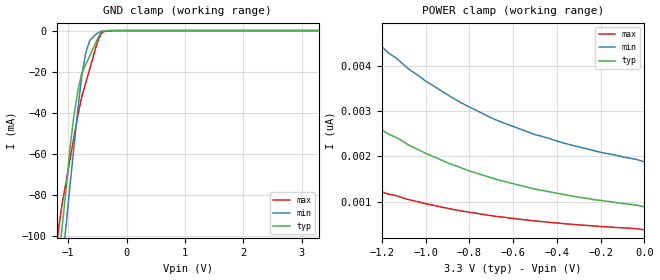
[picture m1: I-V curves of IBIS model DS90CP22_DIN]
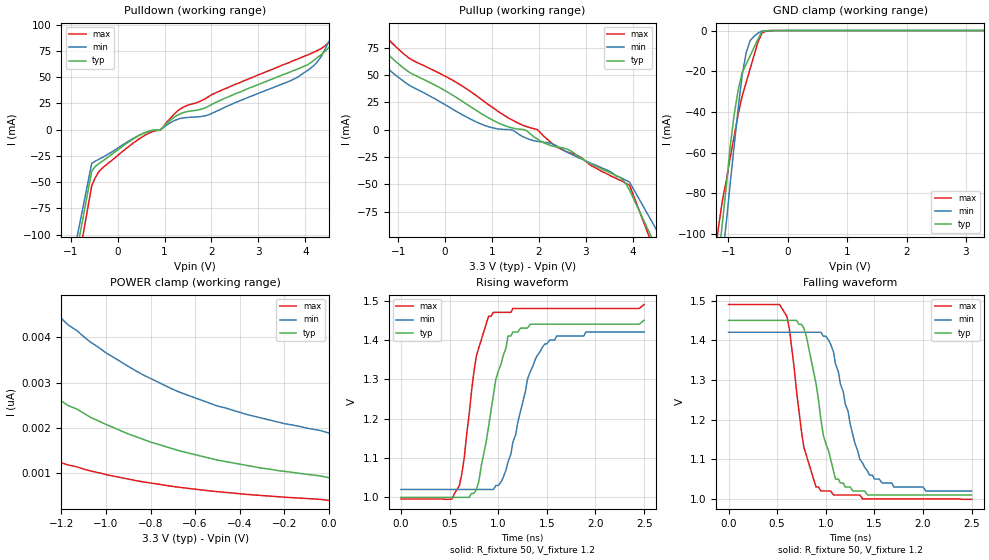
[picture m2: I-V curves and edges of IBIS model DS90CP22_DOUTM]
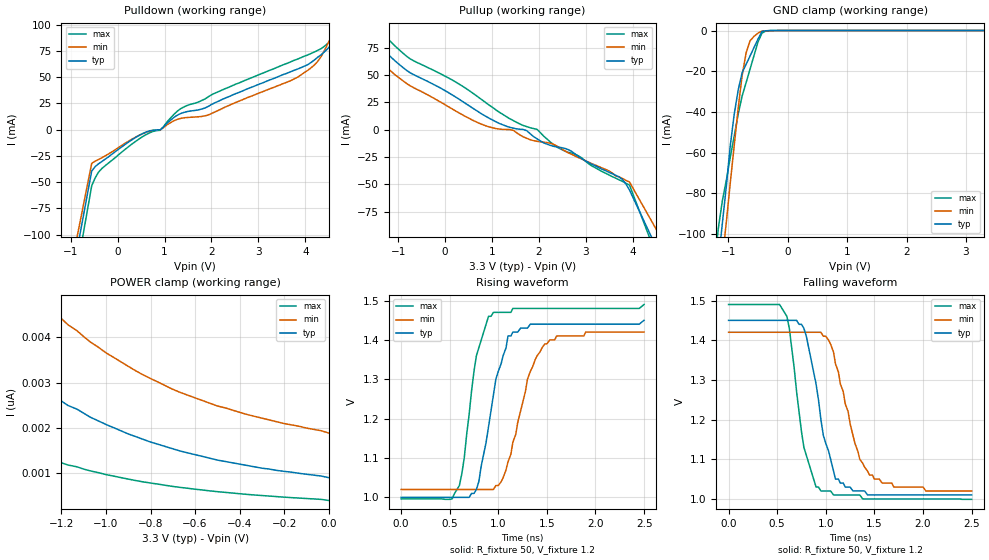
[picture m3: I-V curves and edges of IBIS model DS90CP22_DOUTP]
|   National Semiconductor Corporation
|   IBIS Model of DS90CP22MT
|   2 X 2 800 Mbps LVDS Crosspoint Switch
|   16 Lead TSSOP Package
[IBIS Ver]   3.2
[Comment Char]   |_char
[File name]   ds90cp22mt.ibs
[File Rev]   1.0
[Date]   12/19/03
[Source]
SPICE to IBIS Translation
[Notes]
Created by DG
Rev. 1.0:
- All data from ds90cp22m8 with updated package parasitics for TSSOP package
[Disclaimer]
(C) Copyright National Semiconductor Corporation 2002
   All rights reserved
   National Semiconductor Corporation hereby grants
the user of this IBIS model a non-exclusive, nontransferable
license to use this IBIS model under the following terms.
Before using this IBIS model, the user should read this
license.  If the user does not accept these terms,  the
IBIS model should be returned to National within 30 days.
   The user is granted this license only to use the
IBIS model and is not granted rights to sell, load, rent,
lease or license the IBIS model in whole or in part, or in
modified form to anyone other than user. User may modify
the IBIS model to suit its specific applications but rights
to derivative works and such modifications shall belong to
National.
   This IBIS model is provided on an "AS IS" basis and
National makes absolutely no warranty with respect to the
information contained herein.NATIONAL DISCLAIMS AND CUSTOMER
WAIVES ALL WARRANTIES, EXPRESS OR IMPLIED, INCLUDING
WARRANTIES OF MERCHANTABILITY OR FITNESS FOR A PARTICULAR
PURPOSE. The entire risk as to quality and performance is
with the Customer. ACCORDINGLY, IN NO EVENT SHALL THE
COMPANY BE LIABLE FOR ANY DAMAGES, WHETHER IN CONTRACT OR
TORT,INCLUDING ANY LOST PROFITS OR OTHER INCIDENTAL,
CONSEQUENTIAL, EXEMPLARY, OR PUNITIVE DAMAGES ARISING OUT
OF THE USE OR APPLICATION OF THE IBIS model provided in
this package.Further, National reserves the right to make
changes without notice to any product herein to improve
reliability, function, or design. National does not convey
any license under patent rights or any other intellectual
property rights, including those of third parties.
   National is not obligated to provide maintenance or support
for the licensed IBIS model.
Contact National at ATTN:INTERFACE APPLICATIONS/IBIS MODELS.
5 Foden Road, M/S 03-03, South Porltand, ME 04106
(207) 541-6031
[Copyright]
(c) Copyright 2002 National Semiconductor Corp.
[Component]   DS90CP22MT
Si_location Pin
Timing_location Pin
[Manufacturer]   National Semiconductor Corp.
[Package]
|   TYP   MIN   MAX
R_pkg   91m   78m   115m
L_pkg   2.49n   2.15n   3.12n
C_pkg   0.086p   0.076p   0.109p
[Pin]   signal_name   model_name   R_pin   L_pin   C_pin
1   SEL1   DS90CP22_CONTROL  113m   3.053n   .108p
2   SEL0   DS90CP22_CONTROL   91m   2.494n   .083p
3   IN0+   DS90CP22_DIN   80m   2.218n   .079p
4   IN0-   DS90CP22_DIN   78m   2.157n   .076p
5   VDD   POWER   79m   2.183n   .077p
6   IN1+   DS90CP22_DIN   84m   2.318n   .078p
7   IN1-   DS90CP22_DIN   93m   2.550n   .083p
8   NC   NC   108m   2.984n   .107p
9   NC   NC   115m   3.121n   .109p
10   OUT1-   DS90CP22_DOUTM   93m   2.551n   .083p
11   OUT1+   DS90CP22_DOUTP   81m   2.237n   .079p
12   GND   GND   78m   2.152n   .076p
13   OUT0-   DS90CP22_DOUTM   79m   2.173n   .076p
14   OUT0+   DS90CP22_DOUTP   83m   2.291n   .078p
15   EN1   DS90CP22_CONTROL   90m   2.480n   .083p
16   EN0   DS90CP22_CONTROL  106m   2.914n   .106p
[Diff Pin] inv_pin vdiff   tdelay_typ tdelay_min tdelay_max
| The '+' pin is Diff_pin and the '-' pin is the inv_pin
| Vth/Vtl of Reciever = 100mv
3   4   100mv   0   0   0
6   7   100mv   0   0   0
11   10   0   0   0   0
14   13   0   0   0   0
| Models and submodels in the file (4): DS90CP22_DIN (Input), DS90CP22_DOUTM (3-state), DS90CP22_DOUTP (3-state), DS90CP22_CONTROL (Input)
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[Model]   DS90CP22_DIN
Model_type Input
Vinh=.1
Vinl=-.1
C_comp   2.49pF   2.49pF   2.49pF
[Temperature Range] 25   85   -40
[Voltage Range]   3.3   3.0   3.6
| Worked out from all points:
|   GND clamp passes 1 mA (typ) near -0.44 V on its own axis
[GND Clamp]
|V(groundclamp)   I(typ)   I(min)   I(max)
-3.3V     -803mA     -823mA     -782mA
-1.17V    -114mA     -132mA     -97.7mA
-1.1V     -94.8mA    -112mA     -83.7mA
-1.03V    -75.7mA    -93.4mA    -73.1mA
-967mV    -56.7mA    -75mA      -62.4mA
-900mV    -41.1mA    -56.5mA    -51.8mA
-833mV    -29.2mA    -38.1mA    -41.1mA
-767mV    -20.7mA    -22.1mA    -32.2mA
-700mV    -16.6mA    -11mA      -25.6mA
-633mV    -12.5mA    -5.01mA    -18.9mA
-433mV    -470uA     -263uA     -1.31mA
3.3V      923pA      1.92nA     295pA
[POWER Clamp]
|Vtable   I(typ)   I(min)   I(max)
-3.3V     38.3nA     45.4nA     26.1nA
-2.17V    9.04nA     12.9nA     4.91nA
-2.13V    8.68nA     12.5nA     4.68nA
-2.07V    7.94nA     11.6nA     4.23nA
-1.87V    6.06nA     9.14nA     3.12nA
-1.7V     4.86nA     7.56nA     2.44nA
-1.47V    3.61nA     5.85nA     1.75nA
-1.27V    2.82nA     4.74nA     1.34nA
-1V       2.07nA     3.66nA     958pA
-700mV    1.53nA     2.85nA     695pA
-500mV    1.28nA     2.48nA     579pA
0V        889pA      1.88nA     383pA
[Model]   DS90CP22_DOUTM
Model_type 3-state
Enable Active-High
Polarity Inverting
Vref=1.2
Vmeas=1.2
Rref=50   | 100 Ohms Across Outputs OUTP and OUTM
Cref=5p
C_comp   3.493pF   3.493pF   3.493pF
[Temperature Range] 25   85   -40
[Voltage Range]   3.3   3.0   3.6
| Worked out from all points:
|   slope of the pulldown table from 0 to 0.495 V, typ, clamps not added: 33.8 ohm
|   slope of the pullup table from 0 to 0.495 V, typ, clamps not added: 37.2 ohm
|   GND clamp passes 1 mA (typ) near -0.44 V on its own axis
|   falling waveform, R_fixture 50, V_fixture 1.2: 20-80 % time 212ps typ, 250ps min, 172ps max; typ from 1.45 V to 1.01 V
|   rising waveform, R_fixture 50, V_fixture 1.2: 20-80 % time 217ps typ, 250ps min, 167ps max; typ from 1 V to 1.45 V
[Pullup]
|Vtable   I(typ)   I(min)   I(max)
-3.3V     282mA      249mA      331mA
-1.69V    113mA      101mA      125mA
-1.62V    104mA      93.1mA     115mA
-1.48V    87.5mA     77.5mA     98.1mA
-1.26V    70.3mA     58.2mA     84.4mA
-1.04V    61.8mA     49.2mA     75.3mA
569mV     20.2mA     9.05mA     34mA
1.96V     -8.33mA    -10.6mA    315uA
2.32V     -15.2mA    -13.5mA    -13.9mA
3.56V     -40.2mA    -39.4mA    -42.8mA
3.93V     -55.1mA    -47.8mA    -50.6mA
6.6V      -300mA     -250mA     -350mA
[Pulldown]
|V(pulldown)   I(typ)   I(min)   I(max)
-3.3V     -700mA     -650mA     -750mA
-554mV    -39.4mA    -32mA      -53.4mA
-335mV    -30.2mA    -26.6mA    -36.8mA
468mV     -5.17mA    -5.08mA    -8.42mA
906mV     -142uA     -92.7uA    -509uA
1.34V     15.4mA     10.8mA     20mA
1.93V     22.2mA     14.1mA     31.3mA
3.83V     57.7mA     49.9mA     67.2mA
4.26V     68.9mA     64.9mA     75.5mA
4.7V      94.1mA     103mA      91.8mA
4.85V     110mA      116mA      100mA
6.6V      249mA      159mA      346mA
[GND Clamp]
-3.3V     -803mA     -823mA     -782mA
-1.17V    -114mA     -132mA     -97.7mA
-1.1V     -94.8mA    -112mA     -83.7mA
-1.03V    -75.7mA    -93.4mA    -73.1mA
-967mV    -56.7mA    -75mA      -62.4mA
-900mV    -41.1mA    -56.5mA    -51.8mA
-833mV    -29.2mA    -38.1mA    -41.1mA
-767mV    -20.7mA    -22.1mA    -32.2mA
-700mV    -16.6mA    -11mA      -25.6mA
-633mV    -12.5mA    -5.01mA    -18.9mA
-433mV    -470uA     -263uA     -1.31mA
3.3V      923pA      1.92nA     295pA
[POWER Clamp]
-3.3V     38.3nA     45.4nA     26.1nA
-2.17V    9.04nA     12.9nA     4.91nA
-2.13V    8.68nA     12.5nA     4.68nA
-2.07V    7.94nA     11.6nA     4.23nA
-1.87V    6.06nA     9.14nA     3.12nA
-1.7V     4.86nA     7.56nA     2.44nA
-1.47V    3.61nA     5.85nA     1.75nA
-1.27V    2.82nA     4.74nA     1.34nA
-1V       2.07nA     3.66nA     958pA
-700mV    1.53nA     2.85nA     695pA
-500mV    1.28nA     2.48nA     579pA
0V        889pA      1.88nA     383pA
[Ramp]
dV/dt_r   240mV/.292ns   200mV/.430ns   280mV/.220ns
dV/dt_f   240mv/.300ns   200mv/.400ns   280mv/.220ns
R_load=50
[Falling Waveform]
R_fixture=50
V_fixture=1.2
V_fixture_min=1.2
V_fixture_max=1.2
| Time   V(typ)  V(min)  V(max)
0s        1.45V      1.42V      1.49V
525ps     1.45V      1.42V      1.49V
600ps     1.45V      1.42V      1.46V
775ps     1.43V      1.42V      1.13V
900ps     1.29V      1.42V      1.03V
950ps     1.2V       1.42V      1.02V
1.1ns     1.05V      1.34V      1.01V
1.3ns     1.02V      1.14V      1.01V
1.45ns    1.01V      1.06V      1V
2.5ns     1.01V      1.02V      999mV
[Rising Waveform]
R_fixture=50
V_fixture=1.2
V_fixture_min=1.2
V_fixture_max=1.2
| Time   V(typ)  V(min)  V(max)
0s        1V         1.02V      996mV
525ps     1V         1.02V      996mV
600ps     1V         1.02V      1.03V
650ps     1V         1.02V      1.1V
775ps     1.02V      1.02V      1.36V
950ps     1.26V      1.02V      1.47V
1.1ns     1.41V      1.09V      1.47V
1.3ns     1.43V      1.3V       1.48V
1.48ns    1.44V      1.39V      1.48V
2.5ns     1.45V      1.42V      1.49V
[Model]   DS90CP22_DOUTP
Model_type 3-state
Enable Active-High
Polarity Non-Inverting
Vref=1.2
Vmeas=1.2
Rref=50   | 100 ohms across outputs OUTP and OUTM
Cref=5p
C_comp   3.493pF   3.493pF   3.493pF
[Temperature Range] 25   85   -40
[Voltage Range]   3.3   3.0   3.6
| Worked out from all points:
|   slope of the pulldown table from 0 to 0.495 V, typ, clamps not added: 33.8 ohm
|   slope of the pullup table from 0 to 0.495 V, typ, clamps not added: 37.2 ohm
|   GND clamp passes 1 mA (typ) near -0.44 V on its own axis
|   falling waveform, R_fixture 50, V_fixture 1.2: 20-80 % time 212ps typ, 250ps min, 172ps max; typ from 1.45 V to 1.01 V
|   rising waveform, R_fixture 50, V_fixture 1.2: 20-80 % time 217ps typ, 250ps min, 167ps max; typ from 1 V to 1.45 V
[Pullup]
|Vtable   I(typ)   I(min)   I(max)
-3.3V     282mA      249mA      331mA
-1.69V    113mA      101mA      125mA
-1.62V    104mA      93.1mA     115mA
-1.48V    87.5mA     77.5mA     98.1mA
-1.26V    70.3mA     58.2mA     84.4mA
-1.04V    61.8mA     49.2mA     75.3mA
569mV     20.2mA     9.05mA     34mA
1.96V     -8.33mA    -10.6mA    315uA
2.32V     -15.2mA    -13.5mA    -13.9mA
3.56V     -40.2mA    -39.4mA    -42.8mA
3.93V     -55.1mA    -47.8mA    -50.6mA
6.6V      -300mA     -250mA     -350mA
[Pulldown]
|V(pulldown)   I(typ)   I(min)   I(max)
-3.3V     -700mA     -650mA     -750mA
-554mV    -39.4mA    -32mA      -53.4mA
-335mV    -30.2mA    -26.6mA    -36.8mA
468mV     -5.17mA    -5.08mA    -8.42mA
906mV     -142uA     -92.7uA    -509uA
1.34V     15.4mA     10.8mA     20mA
1.93V     22.2mA     14.1mA     31.3mA
3.83V     57.7mA     49.9mA     67.2mA
4.26V     68.9mA     64.9mA     75.5mA
4.7V      94.1mA     103mA      91.8mA
4.85V     110mA      116mA      100mA
6.6V      249mA      159mA      346mA
[GND Clamp]
-3.3V     -803mA     -823mA     -782mA
-1.17V    -114mA     -132mA     -97.7mA
-1.1V     -94.8mA    -112mA     -83.7mA
-1.03V    -75.7mA    -93.4mA    -73.1mA
-967mV    -56.7mA    -75mA      -62.4mA
-900mV    -41.1mA    -56.5mA    -51.8mA
-833mV    -29.2mA    -38.1mA    -41.1mA
-767mV    -20.7mA    -22.1mA    -32.2mA
-700mV    -16.6mA    -11mA      -25.6mA
-633mV    -12.5mA    -5.01mA    -18.9mA
-433mV    -470uA     -263uA     -1.31mA
3.3V      923pA      1.92nA     295pA
[POWER Clamp]
-3.3V     38.3nA     45.4nA     26.1nA
-2.17V    9.04nA     12.9nA     4.91nA
-2.13V    8.68nA     12.5nA     4.68nA
-2.07V    7.94nA     11.6nA     4.23nA
-1.87V    6.06nA     9.14nA     3.12nA
-1.7V     4.86nA     7.56nA     2.44nA
-1.47V    3.61nA     5.85nA     1.75nA
-1.27V    2.82nA     4.74nA     1.34nA
-1V       2.07nA     3.66nA     958pA
-700mV    1.53nA     2.85nA     695pA
-500mV    1.28nA     2.48nA     579pA
0V        889pA      1.88nA     383pA
[Ramp]
dV/dt_r   240mV/.292ns   200mV/.430ns   280mV/.220ns
dV/dt_f   240mv/.300ns   200mv/.400ns   280mv/.220ns
R_load=50
[Falling Waveform]
R_fixture=50
V_fixture=1.2
V_fixture_min=1.2
V_fixture_max=1.2
| Time   V(typ)  V(min)  V(max)
0s        1.45V      1.42V      1.49V
525ps     1.45V      1.42V      1.49V
600ps     1.45V      1.42V      1.46V
775ps     1.43V      1.42V      1.13V
900ps     1.29V      1.42V      1.03V
950ps     1.2V       1.42V      1.02V
1.1ns     1.05V      1.34V      1.01V
1.3ns     1.02V      1.14V      1.01V
1.45ns    1.01V      1.06V      1V
2.5ns     1.01V      1.02V      999mV
[Rising Waveform]
R_fixture=50
V_fixture=1.2
V_fixture_min=1.2
V_fixture_max=1.2
| Time   V(typ)  V(min)  V(max)
0s        1V         1.02V      996mV
525ps     1V         1.02V      996mV
600ps     1V         1.02V      1.03V
650ps     1V         1.02V      1.1V
775ps     1.02V      1.02V      1.36V
950ps     1.26V      1.02V      1.47V
1.1ns     1.41V      1.09V      1.47V
1.3ns     1.43V      1.3V       1.48V
1.48ns    1.44V      1.39V      1.48V
2.5ns     1.45V      1.42V      1.49V
